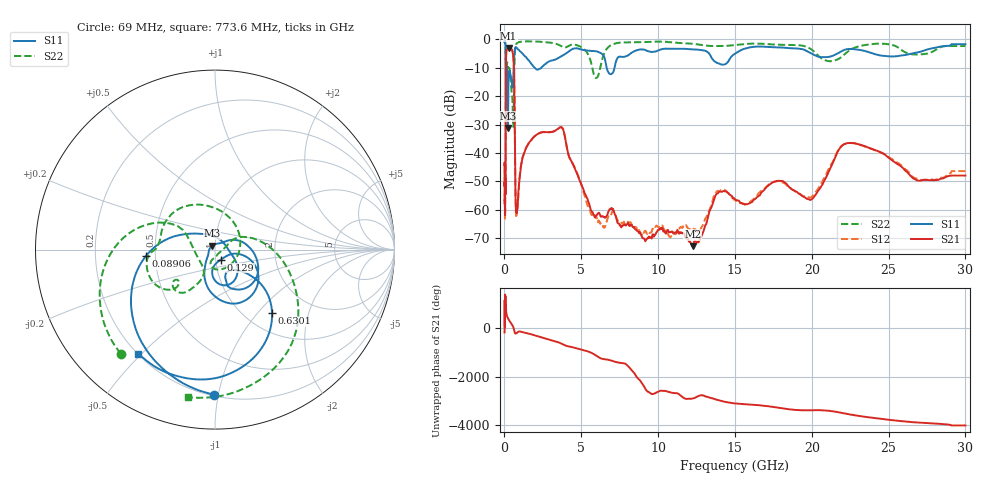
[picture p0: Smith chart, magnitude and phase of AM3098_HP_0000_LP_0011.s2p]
! Date/Time: Thu, Feb 28, 2019 8:30 AM
! Network Analyzer: Agilent Technologies E8364B Rev: A.07.50.67
! Sweep from 0.010 to 30.000 GHz, 1601 Points, Sweep Type: LOG
! Power Supply: 5.023 V, 0.002 A
# Hz S DB R 50
!freq MagS11 AngS11 MagS21 AngS21 MagS12 AngS12 MagS22 AngS22
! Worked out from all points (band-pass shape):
!   1601 points, 10 MHz to 30 GHz, reference 50 ohm
!   highest |S21| = -3.04 dB at 265.1 MHz (marker M1); lowest = -72.9 dB at 12.25 GHz (marker M2)
!   |S21| within 3 dB of the highest: 103.6 MHz to 576.5 MHz (472.9 MHz wide, 139 % of centre)
!   lowest |S11| = -31.2 dB at 227 MHz (marker M3), VSWR 1.06, Z = 48.4 + j2.16 ohm
!   |S11| at or under -10 dB: 175.5 MHz to 598.2 MHz (422.7 MHz wide, 109 % of centre); 1.974 GHz to 2.396 GHz (422.4 MHz wide, 19.3 % of centre); 6.652 GHz to 7.164 GHz (512 MHz wide, 7.41 % of centre)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
!   |S22| runs from -30.8 to -0.5 dB; largest |S21 - S12| = 0.012
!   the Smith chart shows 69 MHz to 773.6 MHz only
!   S11 on the Smith chart (normalised r, x): 69 MHz: 0.21, -0.97; 89.06 MHz: 0.44, -0.04; 129 MHz: 1.06, -0.12; 630.1 MHz: 1.31, -1.20; 773.6 MHz: 0.20, -0.49
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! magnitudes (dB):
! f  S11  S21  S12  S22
! 10 MHz  -0.4  -44.4  -45.0  -0.5
! 38.04 MHz  -0.5  -59.3  -63.3  -0.9
! 69 MHz  -1.9  -52.9  -51.6  -2.1
! 89.06 MHz  -8.2  -18.2  -18.2  -9.9
! 97.94 MHz  -24.2  -7.8  -7.8  -17.6
! 129 MHz  -23.8  -3.9  -3.9  -11.3
! 144.7 MHz  -13.1  -3.6  -3.5  -10.1
! 186.8 MHz  -11.6  -3.5  -3.4  -8.2
! 227 MHz  -31.2  -3.1  -3.1  -9.8
! 265.1 MHz  -14.8  -3.0  -3.0  -10.1
! 550.5 MHz  -15.8  -4.9  -4.9  -27.2
! 630.1 MHz  -6.4  -12.7  -12.7  -13.1
! 773.6 MHz  -2.8  -60.9  -62.6  -1.6
! 2.084 GHz  -10.5  -33.6  -33.6  -0.7
! 3.723 GHz  -5.8  -31.0  -31.0  -2.4
! 5.725 GHz  -4.1  -60.9  -62.1  -10.2
! 7.926 GHz  -5.9  -65.6  -64.0  -1.0
! 12.25 GHz  -3.5  -72.9  -67.2  -1.5
! 14.16 GHz  -8.9  -53.7  -52.9  -2.3
! 19.8 GHz  -4.4  -56.4  -55.8  -3.0
! 22.56 GHz  -3.4  -36.5  -36.5  -3.5
! 30 GHz  -1.7  -48.0  -46.4  -2.3
